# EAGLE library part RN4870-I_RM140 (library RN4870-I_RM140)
Bluetooth Modules (802.15.1) Bluetooth Low Energy BLE Module, Shielded, Antenna, ASCII Interface, 12x22mm Source: Datasheet
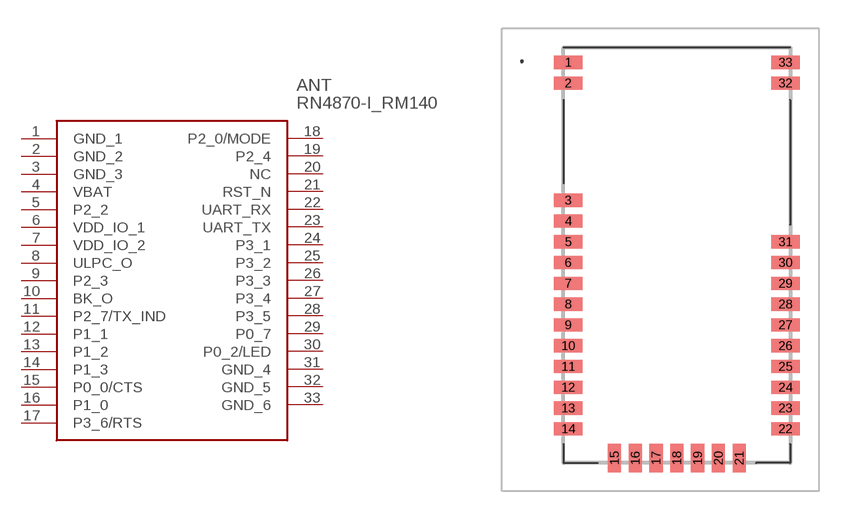
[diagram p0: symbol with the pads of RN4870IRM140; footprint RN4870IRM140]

Designator prefix ANT

## RN4870-I_RM140 (Description: Bluetooth Modules (802.15.1) Bluetooth Low Energy BLE Module, Shielded, Antenna, ASCII Interface, 12x22mm; Height: 2.46mm; Manufacturer_Name: Microchip; Manufacturer_Part_Number: RN4870-I/RM140; Mouser_Part_Number: 579-RN4870-I/RM140; Mouser_Price-Stock: https://www.mouser.co.uk/ProductDetail/Microchip-Technology/RN4870-I-RM140?qs=BJlw7L4Cy7%252BOM7skq4uXXw%3D%3D)  [RN4870IRM140]
1  GND_1
2  GND_2
3  GND_3
4  VBAT
5  P2_2
6  VDD_IO_1
7  VDD_IO_2
8  ULPC_O
9  P2_3
10  BK_O
11  P2_7/TX_IND
12  P1_1
13  P1_2
14  P1_3
15  P0_0/CTS
16  P1_0
17  P3_6/RTS
18  P2_0/MODE
19  P2_4
20  NC  nc
21  RST_N
22  UART_RX
23  UART_TX
24  P3_1
25  P3_2
26  P3_3
27  P3_4
28  P3_5
29  P0_7
30  P0_2/LED
31  GND_4
32  GND_5
33  GND_6

## Footprint RN4870IRM140 (pad centres in mm)
RN4870-I/RM140-4
smd 1.5 x 0.7: 1 -5.75,10.2; 2 -5.75,9.1; 3 -5.75,2.9; 4 -5.75,1.8; 5 -5.75,0.7; 6 -5.75,-0.4; 7 -5.75,-1.5; 8 -5.75,-2.6; 9 -5.75,-3.7; 10 -5.75,-4.8; 11 -5.75,-5.9; 12 -5.75,-7; 13 -5.75,-8.1; 14 -5.75,-9.2; 22 5.75,-9.2; 23 5.75,-8.1; 24 5.75,-7; 25 5.75,-5.9; 26 5.75,-4.8; 27 5.75,-3.7; 28 5.75,-2.6; 29 5.75,-1.5; 30 5.75,-0.4; 31 5.75,0.7; 32 5.75,9.1; 33 5.75,10.2
smd 0.7 x 1.5: 15 -3.3,-10.75; 16 -2.2,-10.75; 17 -1.1,-10.75; 18 0,-10.75; 19 1.1,-10.75; 20 2.2,-10.75; 21 3.3,-10.75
